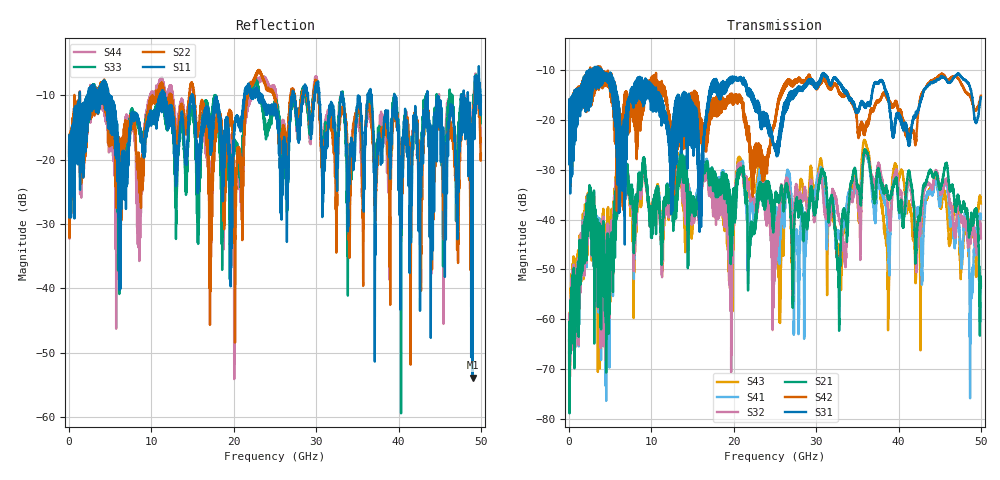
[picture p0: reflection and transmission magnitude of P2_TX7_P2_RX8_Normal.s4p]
!Keysight Technologies,N5225B,MY57041031,A.13.20.10
!Date: Friday, May 31, 2019 11:39:51
!Correction: S11(Full 4 Port(1,2,3,4))
!S12(Full 4 Port(1,2,3,4))
!S13(Full 4 Port(1,2,3,4))
!S14(Full 4 Port(1,2,3,4))
!S21(Full 4 Port(1,2,3,4))
!S22(Full 4 Port(1,2,3,4))
!S23(Full 4 Port(1,2,3,4))
!S24(Full 4 Port(1,2,3,4))
!S31(Full 4 Port(1,2,3,4))
!S32(Full 4 Port(1,2,3,4))
!S33(Full 4 Port(1,2,3,4))
!S34(Full 4 Port(1,2,3,4))
!S41(Full 4 Port(1,2,3,4))
!S42(Full 4 Port(1,2,3,4))
!S43(Full 4 Port(1,2,3,4))
!S44(Full 4 Port(1,2,3,4))
!S4P File: Measurements: <S11,S12,S13,S14>,
!<S21,S22,S23,S24>,
!<S31,S32,S33,S34>,
!<S41,S42,S43,S44>:
# Hz S  dB  R 50.0
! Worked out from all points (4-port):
!   5000 points, 10 MHz to 50 GHz, reference 50 ohm
!   strongest paths, dB at 10 MHz, 12.51 GHz, 25.01 GHz, 37.51 GHz, 50 GHz:
!     S31: -19.6, -22.6, -25.6, -12.7, -15.5
!     S42: -19.5, -21.6, -20.1, -16.3, -15.1
!     S21: -62.1, -37.3, -35.3, -29.8, -53.3
!     S32: -59.0, -37.1, -42.4, -29.2, -43.8
!     S41: -66.7, -36.3, -39.5, -32.8, -39.4
!     S43: -64.2, -35.0, -41.6, -31.9, -36.8
!   lowest |S11| = -53.9 dB at 48.99 GHz (marker M1), VSWR 1.00, Z = 50.1 + j0.193 ohm
!   |S11| at or under -10 dB: 4.911 GHz to 11.03 GHz (6.119 GHz wide, 76.8 % of centre); 14.97 GHz to 21.26 GHz (6.293 GHz wide, 34.7 % of centre); 43.5 GHz to 47.59 GHz (4.083 GHz wide, 8.96 % of centre)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
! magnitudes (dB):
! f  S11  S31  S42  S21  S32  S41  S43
! 10 MHz  -19.5  -19.6  -19.5  -62.1  -59.0  -66.7  -64.2
! 6.2 GHz  -32.5  -24.6  -33.3  -25.1  -25.0  -25.0  -24.8
! 32.73 GHz  -16.3  -12.5  -14.0  -52.6  -39.1  -42.9  -47.5
! 36.03 GHz  -14.5  -17.3  -21.9  -26.5  -26.9  -26.9  -24.6
! 38.67 GHz  -15.2  -14.8  -15.8  -34.9  -36.7  -42.5  -47.3
! 48.99 GHz  -53.9  -16.0  -16.6  -39.8  -40.3  -49.6  -42.5
! 50 GHz  -11.0  -15.5  -15.1  -53.3  -43.8  -39.4  -36.8
